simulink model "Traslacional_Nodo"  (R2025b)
settings: Solver=VariableStepAuto  StartTime=0.0  StopTime=10.0  RelTol=1e-3
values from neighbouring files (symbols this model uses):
  b1 = 4    [Example_Traslacional_Nodo.m]
  b2 = 2    [Example_Traslacional_Nodo.m]
  k = 2    [Example_Traslacional_Nodo.m]
  m = 8    [Example_Traslacional_Nodo.m]

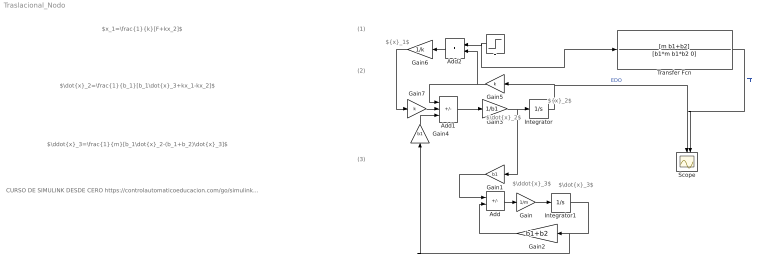
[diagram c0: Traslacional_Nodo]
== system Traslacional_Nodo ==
  note: (3)
  note: (2)
  note: (1)
  note: $\dot{x}_2$
  note: $\ddot{x}_3=\frac{1}{m}[b_1\dot{x}_2-(b_1+b_2)\dot{x}_3]$
  note: $\dot{x}_2=\frac{1}{b_1}[b_1\dot{x}_3+kx_1-kx_2]$
  note: $x_1=\frac{1}{k}[F+kx_2]$
  note: $\ddot{x}_3$
  note: $\dot{x}_3$
  note: ${x}_1$
  note: ${x}_2$
  note: CURSO DE SIMULINK DESDE CERO https://controlautomaticoeducacion.com/go/simulink-cupon/
  Add : Sum  Inputs=+-
  Add1 : Sum  Inputs=-++
  Add2 : Sum
  F : Step  Time=0  SampleTime=0
  Gain : Gain  Gain=1/m
  Gain1 : Gain  Gain=b1
  Gain2 : Gain  Gain=b1+b2
  Gain3 : Gain  Gain=1/b1
  Gain4 : Gain  Gain=b1
  Gain5 : Gain  Gain=k
  Gain6 : Gain  Gain=1/k
  Gain7 : Gain  Gain=k
  Integrator : Integrator
  Integrator1 : Integrator
  Scope : Scope  NumInputPorts=2
  Transfer Fcn : TransferFcn  Numerator=[m b1+b2]  Denominator=[b1*m b1*b2 0]
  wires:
  Integrator1/1 -> Gain4/1, Gain2/1
  Add/1 -> Gain/1
  Gain/1 -> Integrator1/1
  Gain1/1 -> Add/1
  Gain2/1 -> Add/2
  Gain3/1 -> Gain1/1, Integrator/1
  Add1/1 -> Gain3/1
  Gain4/1 -> Add1/3
  Gain5/1 -> Add2/2, Add1/1
  Integrator/1 -> Scope/1, Gain5/1  "EDO"
  F/1 -> Transfer Fcn/1, Add2/1
  Add2/1 -> Gain6/1
  Gain6/1 -> Gain7/1
  Transfer Fcn/1 -> Scope/2  "FT"
  Gain7/1 -> Add1/2
